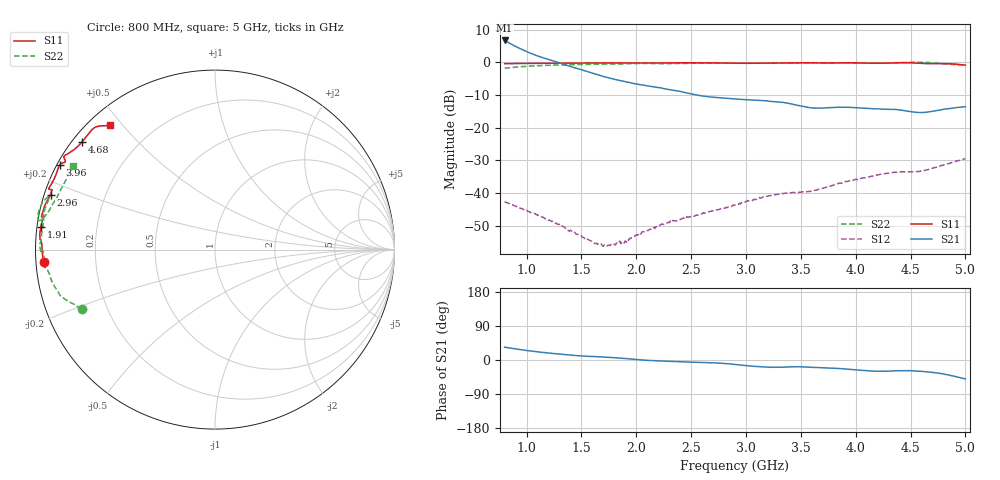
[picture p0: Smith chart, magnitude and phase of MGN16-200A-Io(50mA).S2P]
! Port[1] = GATE
! Port[2] = DRAIN
! [Type]  S-parameter s2p file
! [Object]  MGN16-200A
! [Bias]  50 mA
! [Version]  1.0
! [Date]  Jul 2026
! [Source]  This file was created in JSC "ICC Milandr".
! [Disclaimer] Property of JSC "ICC Milandr". Unauthorized reproduction and/or distribution is strictly prohibited.
!  The file and the data are provided "AS IS" and with all faults and disclaim all warranties, express and implied, including
!  without limitation any implied warranties of merchantability, fitness for a particular purpose.
!  JSC "ICC Milandr" assumes no liability for:
!  1) the accuracy of the data provided;
!  2) the proper functioning of this data;
!  3) infringement of patents, copyrights or intellectual property rights resulting from the use of this data.
!  JSC "ICC Milandr" reserves the right to make changes to the products and the data without prior notice.
!  Please, be aware that your receipt and use of the file provided shall serve as acceptance of these terms and conditions.
!  If you do not accept these terms, you should return or destroy this file and any other accompanying information immediately.
# GHZ S MA R 50
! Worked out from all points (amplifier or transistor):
!   421 points, 800 MHz to 5 GHz, reference 50 ohm
!   highest |S21| = 6.7 dB at 800 MHz (marker M1)
!   |S21| within 3 dB of that: start of sweep to 971.7 MHz
!   unconditionally stable (mu >= 1): 1.446 GHz to 2.198 GHz; 2.208074 GHz to 2.211054 GHz; 4.894 GHz to end of sweep
!   at 1.5 GHz: K = 1.11, MAG = 23.4 dB, |S12| = -53.1 dB
!   at 2.9 GHz: K = 0.56, MSG = 16.2 dB, |S12| = -43.6 dB
!   at 5 GHz: K = 1.68, MAG = 3.1 dB, |S12| = -29.4 dB
!   S11 on the Smith chart (normalised r, x): 800 MHz: 0.02, -0.04; 1.91 GHz: 0.01, +0.06; 2.96 GHz: 0.02, +0.16; 3.96 GHz: 0.01, +0.25; 4.68 GHz: 0.03, +0.36; 5 GHz: 0.06, +0.46
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0.8  0.9553 -175.8  2.159 33.8  0.007416 -43.9  0.8136 -156.1
0.94  0.9613 -178.2  1.623 27.6  0.005907 -47.3  0.8552 -159.7
1.07  0.9639 179.4  1.303 22.7  0.004912 -48.6  0.8824 -162.0
1.21  0.9669 177.7  1.093 18.0  0.003884 -47.9  0.9011 -163.8
1.5  0.9763 176.7  0.7714 10.8  0.002216 -29.0  0.9271 -169.4
1.71  0.9795 175.5  0.6003 7.8  0.00163 4.4  0.9363 -172.4
1.91  0.9777 172.6  0.5007 3.7  0.001777 36.4  0.9495 -173.9
2.2  0.9774 169.3  0.4123 -2.3  0.003216 55.6  0.9564 -176.9
2.38  0.9837 169.2  0.3645 -4.2  0.003885 62.5  0.96 -179.8
2.57  0.9823 168.3  0.3121 -6.3  0.004686 66.5  0.9729 -179.6
2.9  0.9695 162.7  0.2752 -11.7  0.006616 67.8  0.9747 179.4
2.96  0.9662 161.5  0.2708 -13.7  0.007172 66.4  0.9748 178.7
3.18  0.9697 159.9  0.2589 -18.7  0.008905 63.9  0.9687 174.4
3.38  0.9845 160.0  0.2375 -18.4  0.01013 66.8  0.9691 170.1
3.6  0.9827 158.5  0.2006 -19.3  0.01082 67.5  0.9799 171.2
3.77  0.9794 155.3  0.2029 -21.1  0.01284 66.5  0.9756 172.0
3.96  0.9848 151.5  0.205 -24.9  0.01561 63.7  0.9753 169.8
4.3  0.9785 149.0  0.1915 -29.4  0.02017 56.8  0.9679 162.5
4.49  0.9849 147.5  0.1768 -28.1  0.02119 56.6  1.001 166.1
4.68  0.9534 140.9  0.1757 -32.1  0.02355 50.9  0.989 170.6
4.81  0.957 135.4  0.192 -37.5  0.02735 45.7  0.9466 166.3
5  0.9055 130.1  0.2103 -50.0  0.0338 32.9  0.9156 149.5
